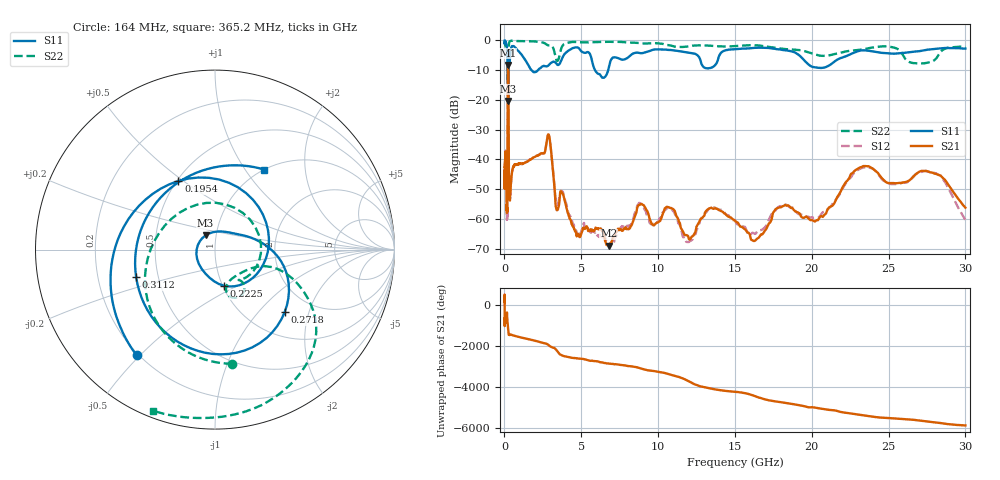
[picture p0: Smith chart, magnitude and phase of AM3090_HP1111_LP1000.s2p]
! Date/Time: Thu, Feb 28, 2019 2:10 PM
! Network Analyzer: Agilent Technologies E8364B Rev: A.07.50.67
! Sweep from 0.010 to 30.000 GHz, 1601 Points, Sweep Type: LOG
! Power Supply: 5.022 V, 0.002 A
# Hz S DB R 50
!freq MagS11 AngS11 MagS21 AngS21 MagS12 AngS12 MagS22 AngS22
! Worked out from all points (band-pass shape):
!   1601 points, 10 MHz to 30 GHz, reference 50 ohm
!   highest |S21| = -8.30 dB at 235.1 MHz (marker M1); lowest = -69.0 dB at 6.787 GHz (marker M2)
!   |S21| within 3 dB of the highest: 214.3 MHz to 254.2 MHz (39.89 MHz wide, 17 % of centre)
!   lowest |S11| = -20.5 dB at 237.5 MHz (marker M3), VSWR 1.21, Z = 44.5 + j7.12 ohm
!   |S11| at or under -10 dB: 207.2 MHz to 257.9 MHz (50.65 MHz wide, 21.8 % of centre); 1.744 GHz to 2.193 GHz (448.1 MHz wide, 22.8 % of centre); 5.885 GHz to 6.756 GHz (870.3 MHz wide, 13.8 % of centre)
!   |S22| runs from -14.6 to -0.1 dB; largest |S21 - S12| = 0.012
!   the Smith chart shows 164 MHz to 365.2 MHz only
!   S11 on the Smith chart (normalised r, x): 164 MHz: 0.19, -0.49; 195.4 MHz: 0.51, +0.48; 222.5 MHz: 1.02, -0.43; 271.8 MHz: 1.47, -1.41; 311.2 MHz: 0.37, -0.15; 365.2 MHz: 1.00, +1.23
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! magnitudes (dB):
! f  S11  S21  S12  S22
! 10 MHz  -0.2  -49.1  -44.8  -0.6
! 38.04 MHz  -0.3  -40.6  -40.5  -1.1
! 98.44 MHz  -0.9  -38.7  -38.9  -3.2
! 144.7 MHz  -1.7  -56.3  -55.9  -3.3
! 164 MHz  -2.7  -56.6  -58.2  -3.8
! 182.2 MHz  -4.7  -55.6  -58.9  -7.6
! 195.4 MHz  -7.3  -36.8  -36.8  -11.8
! 222.5 MHz  -13.6  -9.0  -8.9  -11.9
! 235.1 MHz  -20.3  -8.3  -8.3  -11.4
! 237.5 MHz  -20.5  -8.3  -8.3  -12.2
! 271.8 MHz  -5.6  -28.4  -28.4  -4.7
! 311.2 MHz  -6.6  -52.6  -50.9  -0.7
! 365.2 MHz  -5.6  -53.4  -53.1  -0.3
! 550.5 MHz  -2.0  -42.7  -43.2  -0.2
! 2.084 GHz  -10.6  -38.8  -38.8  -0.5
! 2.884 GHz  -8.4  -31.8  -31.7  -1.8
! 3.419 GHz  -8.1  -57.1  -55.2  -7.0
! 6.787 GHz  -9.3  -69.0  -69.1  -0.6
! 7.926 GHz  -6.2  -63.4  -62.7  -0.8
! 16.46 GHz  -2.6  -66.6  -64.1  -1.8
! 23.48 GHz  -3.4  -42.3  -42.7  -3.0
! 30 GHz  -2.8  -56.2  -60.4  -2.2
